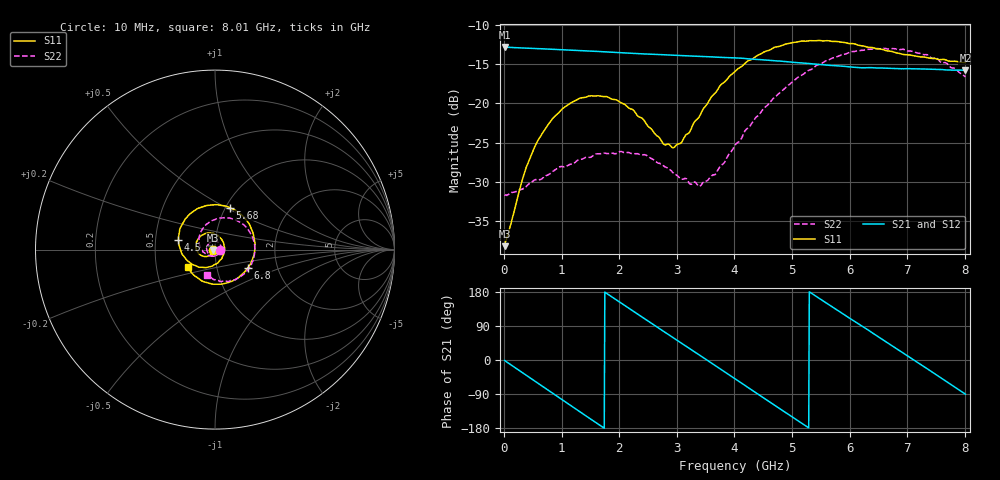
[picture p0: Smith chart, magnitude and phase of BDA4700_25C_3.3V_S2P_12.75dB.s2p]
!Agilent Technologies,E5071B,MY42404982,A.09.10
!Date: Mon Oct 20 18:08:23 2025
!Data & Calibration Information:
!Freq	S11:SOLT2(ON)	S21:SOLT2(ON)	S12:SOLT2(ON)	S22:SOLT2(ON)
# Hz S RI R 50
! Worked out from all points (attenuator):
!   801 points, 10 MHz to 8.01 GHz, reference 50 ohm
!   highest |S21| = -12.85 dB at 10 MHz (marker M1); lowest = -15.8 dB at 8.01 GHz (marker M2)
!   lowest |S11| = -38.2 dB at 10 MHz (marker M3), VSWR 1.03, Z = 48.8 - j0.154 ohm
!   |S11| at or under -10 dB: start of sweep to end of sweep
!   |S22| runs from -31.7 to -13.0 dB; largest |S21 - S12| = 0.0027
!   S11 on the Smith chart (normalised r, x): 10 MHz: 0.98, -0.00; 4.5 GHz: 0.66, +0.07; 5.68 GHz: 1.04, +0.52; 6.8 GHz: 1.41, -0.30; 8.01 GHz: 0.72, -0.15
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1e7  -0.0123 -0.00158  0.2277 -0.00494  0.2276 -0.00518  0.0262 -0.000945
3.5e8  -0.0235 -0.0269  0.1793 -0.1345  0.1792 -0.1346  0.0223 -0.0183
5.7e8  -0.0419 -0.0379  0.1123 -0.1921  0.112 -0.1921  0.0141 -0.0296
8.7e8  -0.0744 -0.034  -0.0026 -0.2199  -0.0025 -0.22  -0.00858 -0.0364
1.35e9  -0.1069 0.0176  -0.1655 -0.1386  -0.1655 -0.1386  -0.0415 -0.015
1.64e9  -0.0945 0.0593  -0.2098 -0.0379  -0.2098 -0.038  -0.0466 0.0104
1.94e9  -0.0571 0.0885  -0.1971 0.0733  -0.1972 0.0732  -0.0328 0.0349
2.33e9  0.00653 0.0823  -0.1037 0.1788  -0.1036 0.1788  -0.00118 0.0476
2.68e9  0.0474 0.0388  0.0187 0.203  0.0183 0.2029  0.0256 0.0329
2.96e9  0.0507 -0.0142  0.111 0.1682  0.1108 0.1679  0.0338 0.0112
3.4e9  -0.00216 -0.0834  0.194 0.042  0.1942 0.0421  0.0176 -0.024
3.67e9  -0.0612 -0.0992  0.1898 -0.0509  0.1898 -0.0514  -0.00662 -0.0349
4.01e9  -0.1425 -0.0708  0.1259 -0.1478  0.1261 -0.1474  -0.0453 -0.0288
4.5e9  -0.2038 0.0521  -0.0306 -0.1861  -0.0303 -0.1865  -0.087 0.0286
4.94e9  -0.1566 0.1816  -0.148 -0.1081  -0.1478 -0.109  -0.0744 0.1074
5.35e9  -0.0345 0.2471  -0.1772 0.016  -0.1774 0.0148  -0.0056 0.165
5.68e9  0.0811 0.2341  -0.1371 0.1068  -0.1371 0.1069  0.0764 0.1762
6.21e9  0.2091 0.0995  -0.000348 0.1681  0.00203 0.1685  0.1936 0.0979
6.68e9  0.2046 -0.0648  0.1211 0.1144  0.1215 0.1143  0.2195 -0.0275
6.8e9  0.1831 -0.1019  0.1415 0.0871  0.1421 0.0861  0.2133 -0.0591
7.37e9  0.018 -0.193  0.1489 -0.0706  0.1489 -0.0706  0.1109 -0.1691
8.01e9  -0.1523 -0.0989  -0.000359 -0.1618  0.000193 -0.162  -0.0462 -0.1394
